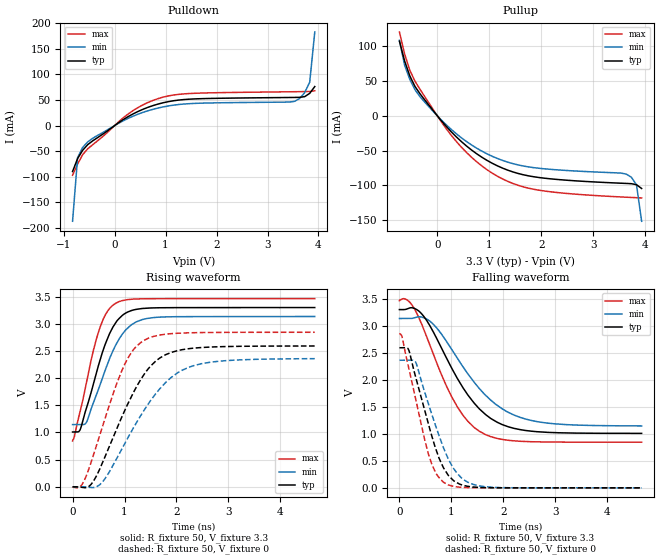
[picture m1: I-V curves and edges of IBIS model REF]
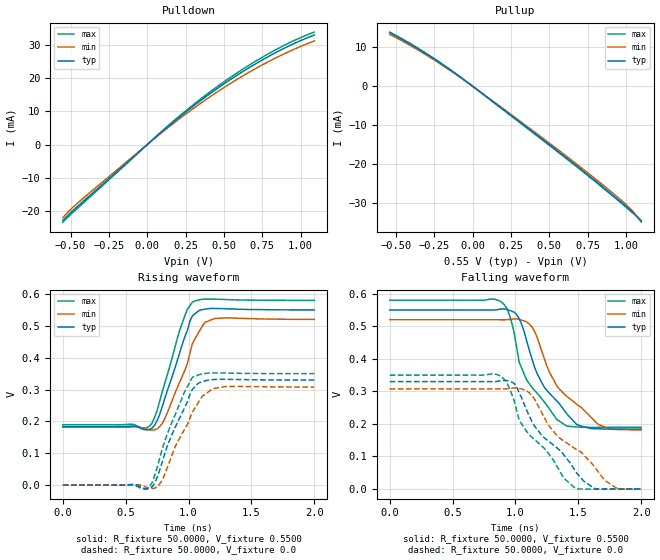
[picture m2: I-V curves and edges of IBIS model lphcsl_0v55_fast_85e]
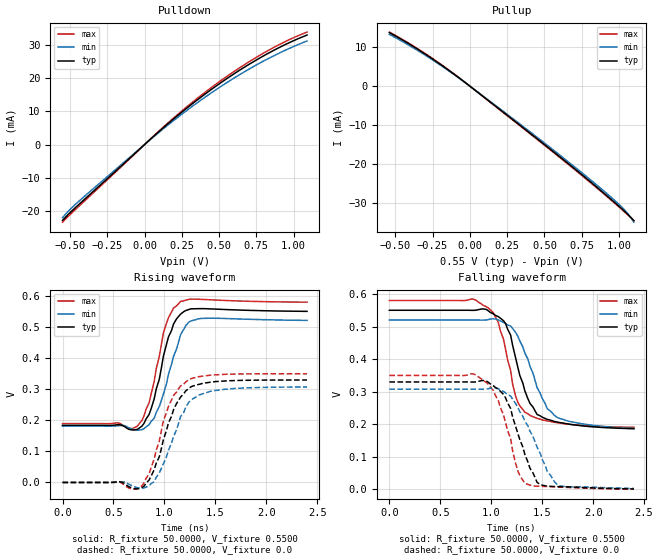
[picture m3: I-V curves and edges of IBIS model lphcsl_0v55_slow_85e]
| Integrated Devices Technolgy, Inc
[IBIS Ver]   4.1
[File name]   9fgl0651.ibs
[File Rev]   1.0
|Rev history   1.0   original ibis data
[Date]   30 March, 2016
[Disclaimer] Integrated Device Technology, Inc. ("IDT") hereby grants the
   user of this ibis model a non-exclusive, nontransferable
   license to use this ibis model under the following terms. the
   user is granted this license only to use the ibis model and is
   not granted rights to sell, copy (except as needed to run the
   ibis model), rent, lease or sub-license the ibis model in
   whole or in part, or in modified form to anyone. the user may
   modify the ibis model to suit its specific applications, but
   rights to derivative works and such modifications shall belong
   to idt. this ibis model is provided on an as is" basis and idt
   makes absolutely no warranty with respect to the information
   contained herein. idt disclaims and customer waives all
   warranties, express and implied, including warranties of
   merchantability and fitness for a particular purpose. the
   entire risk as to quality and performance is with the user
   accordingly, in no event shall idt be liable for any direct or
   indirect damages, whether in contract or tort, including any
   lost profits or other incidental, consequential, exemplary, or
   punitive damages arising out of the use or application of the
   ibis model. further, idt reserves the right to make changes
   without notice to any product herein to improve reliability,
   function, or design. idt does not convey any license under
   patent rights or any other intellectual property rights,
   including those of third parties. idt is not obligated to
   provide maintenance or support for the licensed ibis model.
[Copyright]   Copyright 2012, Integrated Devices Technolgy, Inc. all rights
   reserved
[Component]   9fgl0651
[Manufacturer] Integrated Device Technology, Inc.
[Package]
R_pkg   72.4655m   58.886m   86.045m
L_pkg   1.47175nH   1.11650nH   1.77850nH
C_pkg   0.07747pF   0.07444pF   0.08050pF
[Pin] signal_name  model_name
1   vSS_EN_tri   GND
2   X1_25   X1
3   X2   X2
4   VDDXTAL3.3   POWER
5   VDDREF3.3   POWER
6   vSADR/REF3.3   REF
7   NC   NC
8   GNDDIG   GND
9   SCLK_3.3   SCIN
10   SDATA_3.3   SCIN
11   VDDDIG3.3   POWER
12   VDDIO   POWER
13   vOE0#   IN
14   DIF0   LP_HCSL
15   DIF0#   LP_HCSL
16   VDD3.3   POWER
17   VDDIO   POWER
18   DIF1   LP_HCSL
19   DIF1#   LP_HCSL
20   NC   NC
21   vOE1#   IN
22   DIF2   LP_HCSL
23   DIF2#   LP_HCSL
24   vOE2#   IN
25   NC   NC
26   VDDA3.3   POWER
27   VDDIO   POWER
28   DIF3   LP_HCSL
29   DIF3#   LP_HCSL
30   vOE3#   IN
31   VDD3.3   POWER
32   VDDIO   POWER
33   DIF4   LP_HCSL
34   DIF4#   LP_HCSL
35   vOE4#   IN
36   DIF5   LP_HCSL
37   DIF5#   LP_HCSL
38   vOE5#   IN
39   VDDIO   POWER
40   ^CKPWRGD_PD#   PD
41   ePAD   GND
[Diff Pin]  inv_pin  vdiff tdelay_typ tdelay_min  tdelay_max
14   15   NA   0   0   0
18   19   NA   0   0   0
22   23   NA   0   0   0
28   29   NA   0   0   0
33   34   NA   0   0   0
36   37   NA   0   0   0
[Model Selector] LP_HCSL
lphcsl_0v55_fast_85e amplitude 0.55V, slew rate fast
lphcsl_0v55_slow_85e amplitude 0.55V, slew rate slow
lphcsl_0v65_fast_85e amplitude 0.65V, slew rate fast
lphcsl_0v65_slow_85e amplitude 0.65V, slew rate slow
lphcsl_0v70_fast_85e amplitude 0.70V, slew rate fast
lphcsl_0v70_slow_85e amplitude 0.70V, slew rate slow
lphcsl_0v80_fast_85e amplitude 0.80V, slew rate fast
lphcsl_0v80_slow_85e amplitude 0.80V, slew rate slow
| Models and submodels in the file (14): REF (Output), lphcsl_0v55_fast_85e (Output), lphcsl_0v55_slow_85e (Output), lphcsl_0v65_fast_85e (Output), lphcsl_0v65_slow_85e (Output), lphcsl_0v70_fast_85e (Output), lphcsl_0v70_slow_85e (Output), lphcsl_0v80_fast_85e (Output), lphcsl_0v80_slow_85e (Output), SCIN (Input), IN (Input), PD (Input), X1 (Input), X2 (Output)
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[Model]   REF
Model_type   Output
Polarity   Non-Inverting
|   typ   min   max
C_comp   2pF   1.5pF   2.5pF
Vmeas = 1.65V
Rref = 50
Cref = 0
Vref = 1.65V
|   typ   min   max
[Voltage range]   3.3V   3.135V   3.465V
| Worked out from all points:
|   slope of the pulldown table from 0 to 0.495 V, typ, clamps not added: 16.9 ohm
|   slope of the pullup table from 0 to 0.495 V, typ, clamps not added: 12.6 ohm
|   rising waveform, R_fixture 50, V_fixture 3.3: 20-80 % time 450ps typ, 507ps min, 388ps max; typ from 1.01 V to 3.3 V
|   falling waveform, R_fixture 50, V_fixture 3.3: 20-80 % time 857ps typ, 970ps min, 739ps max; typ from 3.3 V to 1.01 V
|   rising waveform, R_fixture 50, V_fixture 0: 20-80 % time 771ps typ, 936ps min, 618ps max; typ from 0 V to 2.59 V
|   falling waveform, R_fixture 50, V_fixture 0: 20-80 % time 472ps typ, 527ps min, 413ps max; typ from 2.59 V to 0 V
[Pulldown]
|Voltage   I (typ)   I (min)   I (max)
|Note, modeling breaks down at 250mA and above.  This is well beyond the functional   |
|operating range of the device.  Should this scenario occur, catastrophic failure and   |
|possible damage to the device and/or board is of higher concern than the I-V curve   |
|behavior.  The IBIS checker will flag currents in excess of 10A with warnings.  Lines   |
|with currents in excess of 0.35 A have been commented out.  The points still remain|
|available to the user if the user desires to use them.   |
|-3.30000e+00   -4.58626e+02   -3.98855e+02   -5.58913e+02
|-3.20100e+00   -4.38670e+02   -3.81813e+02   -5.34126e+02
|-3.10200e+00   -4.18718e+02   -3.64776e+02   -5.09343e+02
|-3.00300e+00   -3.98770e+02   -3.47745e+02   -4.84563e+02
|-2.90400e+00   -3.78827e+02   -3.30720e+02   -4.59787e+02
|-2.80500e+00   -3.58890e+02   -3.13701e+02   -4.35015e+02
|-2.70600e+00   -3.38959e+02   -2.96690e+02   -4.10248e+02
|-2.60700e+00   -3.19035e+02   -2.79688e+02   -3.85486e+02
|-2.50800e+00   -2.99119e+02   -2.62696e+02   -3.60731e+02
|-2.40900e+00   -2.79213e+02   -2.45715e+02   -3.35984e+02
|-2.31000e+00   -2.59319e+02   -2.28747e+02   -3.11245e+02
|-2.21100e+00   -2.39437e+02   -2.11796e+02   -2.86516e+02
|-2.11200e+00   -2.19572e+02   -1.94864e+02   -2.61800e+02
|-2.01300e+00   -1.99726e+02   -1.77955e+02   -2.37100e+02
|-1.91400e+00   -1.79905e+02   -1.61075e+02   -2.12419e+02
|-1.81500e+00   -1.60116e+02   -1.44233e+02   -1.87763e+02
|-1.71600e+00   -1.40369e+02   -1.27441e+02   -1.63140e+02
|-1.61700e+00   -1.20682e+02   -1.10717e+02   -1.38565e+02
|-1.51800e+00   -1.01080e+02   -9.40899e+01   -1.14061e+02
|-1.41900e+00   -8.16135e+01   -7.76121e+01   -8.96701e+01
|-1.32000e+00   -6.23864e+01   -6.13830e+01   -6.54941e+01
|-1.22100e+00   -4.36066e+01   -4.55730e+01   -4.17841e+01
|-1.12200e+00   -2.55446e+01   -3.03740e+01   -1.89497e+01
|-1.02300e+00   -8.13369e+00   -1.57511e+01   -1.01906e+00
|-9.24000e-01   -3.55892e-01   -2.38948e+00   -1.27879e-01
-825mV    -89.74mA   -186.9mA   -97.05mA
-726mV    -64.34mA   -62.46mA   -75.03mA
-627mV    -48.3mA    -42.65mA   -56.86mA
-528mV    -37.22mA   -31.89mA   -45.33mA
363mV     22.88mA    18.45mA    29.33mA
957mV     44.74mA    36.62mA    55.73mA
1.551V    52.05mA    43.3mA     63.04mA
3.531V    55.03mA    47.39mA    66.19mA
3.63V     55.21mA    52.95mA    66.32mA
3.729V    56.59mA    64.36mA    66.46mA
3.828V    63.02mA    84.81mA    66.64mA
3.927V    76.26mA    182.8mA    67.99mA
| 4.02600e+00   9.63336e-02   1.95544e+00   7.56685e-02
| 4.12500e+00   1.29319e-01   1.96109e+01   9.19025e-02
| 4.22400e+00   6.62462e-01   4.21550e+01   1.15435e-01
| 4.32300e+00   1.51637e+01   6.47670e+01   1.37492e-01
| 4.42200e+00   4.22442e+01   8.74545e+01   2.35006e-01
| 4.52100e+00   6.94172e+01   1.10195e+02   8.92943e+00
| 4.62000e+00   9.66780e+01   1.32968e+02   4.35589e+01
| 4.71900e+00   1.23991e+02   1.55761e+02   7.83218e+01
| 4.81800e+00   1.51333e+02   1.78569e+02   1.13180e+02
| 4.91700e+00   1.78693e+02   2.01386e+02   1.48085e+02
| 5.01600e+00   2.06065e+02   2.24210e+02   1.83014e+02
| 5.11500e+00   2.33446e+02   2.47041e+02   2.17958e+02
| 5.21400e+00   2.60834e+02   2.69877e+02   2.52912e+02
| 5.31300e+00   2.88228e+02   2.92717e+02   2.87874e+02
| 5.41200e+00   3.15625e+02   3.15560e+02   3.22841e+02
| 5.51100e+00   3.43027e+02   3.38407e+02   3.57813e+02
| 5.61000e+00   3.70432e+02   3.61256e+02   3.92789e+02
| 5.70900e+00   3.97841e+02   3.84108e+02   4.27769e+02
| 5.80800e+00   4.25252e+02   4.06963e+02   4.62752e+02
| 5.90700e+00   4.52666e+02   4.29821e+02   4.97738e+02
| 6.00600e+00   4.80082e+02   4.52680e+02   5.32727e+02
| 6.10500e+00   5.07501e+02   4.75543e+02   5.67718e+02
| 6.20400e+00   5.34922e+02   4.98407e+02   6.02711e+02
| 6.30300e+00   5.62345e+02   5.21273e+02   6.37705e+02
| 6.40200e+00   5.89770e+02   5.44142e+02   6.72701e+02
| 6.50100e+00   6.17197e+02   5.67013e+02   7.07699e+02
| 6.60000e+00   6.44626e+02   5.89886e+02   7.42698e+02
[Pullup]
|Voltage   I (typ)   I (min)   I (max)
|Note, modeling breaks down at 250mA and above.  This is well beyond the functional   |
|operating range of the device.  Should this scenario occur, catastrophic failure and   |
|possible damage to the device and/or board is of higher concern than the I-V curve   |
|behavior.  The IBIS checker will flag currents in excess of 10A with warnings.  Lines   |
|with currents in excess of 0.35 A have been commented out.  The points still remain|
|available to the user if the user desires to use them.   |
|-3.30000e+00   6.44680e+02   5.51825e+02   8.01095e+02
|-3.20100e+00   6.17254e+02   5.28958e+02   7.66095e+02
|-3.10200e+00   5.89830e+02   5.06093e+02   7.31096e+02
|-3.00300e+00   5.62407e+02   4.83230e+02   6.96098e+02
|-2.90400e+00   5.34987e+02   4.60368e+02   6.61102e+02
|-2.80500e+00   5.07568e+02   4.37509e+02   6.26108e+02
|-2.70600e+00   4.80150e+02   4.14651e+02   5.91115e+02
|-2.60700e+00   4.52735e+02   3.91796e+02   5.56124e+02
|-2.50800e+00   4.25322e+02   3.68942e+02   5.21136e+02
|-2.40900e+00   3.97911e+02   3.46091e+02   4.86149e+02
|-2.31000e+00   3.70503e+02   3.23243e+02   4.51165e+02
|-2.21100e+00   3.43097e+02   3.00397e+02   4.16183e+02
|-2.11200e+00   3.15694e+02   2.77554e+02   3.81204e+02
|-2.01300e+00   2.88295e+02   2.54715e+02   3.46229e+02
|-1.91400e+00   2.60900e+02   2.31881e+02   3.11257e+02
|-1.81500e+00   2.33510e+02   2.09052e+02   2.76290e+02
|-1.71600e+00   2.06127e+02   1.86229e+02   2.41329e+02
|-1.61700e+00   1.78751e+02   1.63415e+02   2.06375e+02
|-1.51800e+00   1.51388e+02   1.40613e+02   1.71432e+02
|-1.41900e+00   1.24042e+02   1.17829e+02   1.36506e+02
|-1.32000e+00   9.67252e+01   9.50724e+01   1.01609e+02
|-1.22100e+00   6.94599e+01   7.23604e+01   6.67700e+01
|-1.12200e+00   4.22820e+01   4.97173e+01   3.20469e+01
|-1.02300e+00   1.51962e+01   2.71494e+01   2.11287e+00
|-9.24000e-01   6.89030e-01   5.34223e+00   1.97623e-01
|-8.25000e-01   1.48916e-01   3.54714e-01   1.54087e-01
-726mV    106.9mA    108.2mA    120.1mA
-627mV    78.63mA    72.64mA    88.74mA
-528mV    57.36mA    52.3mA     65.5mA
-330mV    31.45mA    27.24mA    37.82mA
363mV     -30.02mA   -25.58mA   -36.52mA
957mV     -64.05mA   -54.65mA   -77.43mA
1.353V    -77.99mA   -66.51mA   -94.06mA
1.848V    -87.45mA   -74.38mA   -105.4mA
3.63V     -97.08mA   -83.63mA   -116.9mA
3.729V    -97.47mA   -88.18mA   -117.2mA
3.828V    -98.9mA    -99mA      -117.5mA
3.927V    -104.4mA   -151.4mA   -117.9mA
| 4.02600e+00   -1.15410e-01   -9.65481e-01   -1.19366e-01
| 4.12500e+00   -1.36603e-01   -1.09884e+01   -1.26324e-01
| 4.22400e+00   -3.99361e-01   -2.54841e+01   -1.40663e-01
| 4.32300e+00   -8.17474e+00   -4.04654e+01   -1.58277e-01
| 4.42200e+00   -2.55843e+01   -5.60873e+01   -2.17491e-01
| 4.52100e+00   -4.36450e+01   -7.21990e+01   -4.28595e+00
| 4.62000e+00   -6.24226e+01   -8.86071e+01   -2.64922e+01
| 4.71900e+00   -8.16508e+01   -1.05189e+02   -4.96573e+01
| 4.81800e+00   -1.01115e+02   -1.21884e+02   -7.35635e+01
| 4.91700e+00   -1.20715e+02   -1.38656e+02   -9.78285e+01
| 5.01600e+00   -1.40403e+02   -1.55482e+02   -1.22263e+02
| 5.11500e+00   -1.60149e+02   -1.72350e+02   -1.46794e+02
| 5.21400e+00   -1.79938e+02   -1.89250e+02   -1.71387e+02
| 5.31300e+00   -1.99760e+02   -2.06175e+02   -1.96022e+02
| 5.41200e+00   -2.19606e+02   -2.23121e+02   -2.20688e+02
| 5.51100e+00   -2.39472e+02   -2.40084e+02   -2.45378e+02
| 5.61000e+00   -2.59355e+02   -2.57061e+02   -2.70086e+02
| 5.70900e+00   -2.79251e+02   -2.74051e+02   -2.94808e+02
| 5.80800e+00   -2.99159e+02   -2.91052e+02   -3.19543e+02
| 5.90700e+00   -3.19077e+02   -3.08062e+02   -3.44288e+02
| 6.00600e+00   -3.39003e+02   -3.25080e+02   -3.69042e+02
| 6.10500e+00   -3.58937e+02   -3.42106e+02   -3.93803e+02
| 6.20400e+00   -3.78878e+02   -3.59138e+02   -4.18571e+02
| 6.30300e+00   -3.98826e+02   -3.76177e+02   -4.43346e+02
| 6.40200e+00   -4.18779e+02   -3.93221e+02   -4.68125e+02
| 6.50100e+00   -4.38737e+02   -4.10271e+02   -4.92910e+02
| 6.60000e+00   -4.58699e+02   -4.27325e+02   -5.17700e+02
[Ramp]
|   typ   min   max
dV/dt_r   1.566/0.774n   1.425/0.94n   1.718/0.621n
dV/dt_f   1.396/0.866n   1.212/0.979n   1.595/0.746n
R_load =   50
[Rising Waveform]
R_fixture = 50
V_fixture = 3.3   |Vcc_typ
V_fixture_min = 3.135 |Vcc_min
V_fixture_max = 3.465 |Vcc_max
C_fixture = 0.0p
| Time   typ   min   max
0s        1.008V     1.145V     844.6mV
34.71ps   1.008V     1.145V     923.1mV
154.3ps   1.071V     1.145V     1.413V
275.2ps   1.472V     1.202V     1.956V
479.5ps   2.168V     1.745V     2.789V
635.5ps   2.641V     2.166V     3.174V
823.7ps   3.01V      2.596V     3.375V
1.129ns   3.244V     2.981V     3.453V
1.433ns   3.289V     3.099V     3.463V
4.662ns   3.3V       3.135V     3.465V
[Falling Waveform]
R_fixture = 50
V_fixture = 3.3   |Vcc_typ
V_fixture_min = 3.135 |Vcc_min
V_fixture_max = 3.465 |Vcc_max
C_fixture = 0.0p
| Time   typ   min   max
0s        3.3V       3.135V     3.465V
120.3ps   3.304V     3.135V     3.493V
247.8ps   3.333V     3.138V     3.377V
425ps     3.225V     3.162V     3.038V
624.4ps   2.937V     3.054V     2.545V
1.111ns   2.034V     2.407V     1.506V
1.539ns   1.462V     1.838V     1.048V
1.979ns   1.171V     1.463V     896.3mV
2.515ns   1.052V     1.252V     854.4mV
4.666ns   1.008V     1.146V     844.6mV
[Rising Waveform]
R_fixture = 50
V_fixture = 0
C_fixture = 0.0p
| Time   typ   min   max
0s        23.89nV    60.43nV    30.4nV
191.1ps   -13.44mV   129.7uV    54.48mV
415.8ps   124mV      -13.01mV   625.4mV
623.1ps   548.9mV    147.1mV    1.254V
939.4ps   1.267V     680mV      2.117V
1.156ns   1.708V     1.059V     2.505V
1.348ns   2.027V     1.367V     2.681V
1.787ns   2.43V      1.916V     2.809V
2.339ns   2.554V     2.232V     2.838V
4.662ns   2.593V     2.359V     2.845V
[Falling Waveform]
R_fixture = 50
V_fixture = 0
C_fixture = 0.0p
| Time   typ   min   max
0s        2.593V     2.362V     2.845V
47.92ps   2.593V     2.362V     2.804V
169.8ps   2.571V     2.362V     2.258V
309ps     2.063V     2.332V     1.656V
482.9ps   1.445V     1.783V     905.2mV
624.2ps   958.6mV    1.36V      434.3mV
847.8ps   371.4mV    743.3mV    103.8mV
1.113ns   93.12mV    264.4mV    16.96mV
1.53ns    8.102mV    37.41mV    1.012mV
4.662ns   -1.039uV   -794nV     -867.7nV
[Model]   lphcsl_0v55_fast_85e
Model_type Output
Polarity   Inverting
Enable   Active-High
Vmeas =  0.4000V
Cref =   2.0000pF
Rref =   0.0
Vref =   0.4000V
C_comp   1.1000pF   1.0000pF   1.2000pF
[Temperature Range]   25.0000   85.0000   -40.0
[Voltage Range]   0.5500V   0.5200V   0.5800V
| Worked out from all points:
|   slope of the pulldown table from 0 to 0.083 V, typ, clamps not added: 24.5 ohm
|   slope of the pullup table from 0 to 0.083 V, typ, clamps not added: 33.4 ohm
|   rising waveform, R_fixture 50.0000, V_fixture 0.5500: 20-80 % time 183ps typ, 188ps min, 171ps max; typ from 0.184 V to 0.55 V
|   rising waveform, R_fixture 50.0000, V_fixture 0.0: 20-80 % time 207ps typ, 220ps min, 194ps max; typ from 0 V to 0.33 V
|   falling waveform, R_fixture 50.0000, V_fixture 0.5500: 20-80 % time 284ps typ, 342ps min, 253ps max; typ from 0.55 V to 0.184 V
|   falling waveform, R_fixture 50.0000, V_fixture 0.0: 20-80 % time 393ps typ, 449ps min, 348ps max; typ from 0.33 V to 0 V
[Pulldown]
|Voltage   I(typ)   I(min)   I(max)
-550mV    -22.86mA   -22.05mA   -23.4mA
-490mV    -20.12mA   -19.14mA   -20.7mA
-430mV    -17.63mA   -16.68mA   -18.17mA
50mV      2.058mA    1.922mA    2.135mA
230mV     9.045mA    8.465mA    9.373mA
410mV     15.37mA    14.42mA    15.91mA
590mV     21.04mA    19.77mA    21.74mA
770mV     26.03mA    24.5mA     26.86mA
930mV     29.87mA    28.16mA    30.76mA
1.09V     33.04mA    31.25mA    33.93mA
[Pullup]
|Voltage   I(typ)   I(min)   I(max)
-540mV    13.79mA    13.35mA    13.94mA
-360mV    9.757mA    9.424mA    9.891mA
-180mV    5.143mA    4.956mA    5.227mA
-20mV     596.4uA    573.5uA    607.4uA
340mV     -10.2mA    -9.898mA   -10.34mA
640mV     -19.35mA   -18.88mA   -19.54mA
920mV     -28.28mA   -27.72mA   -28.48mA
1.04V     -32.36mA   -32.02mA   -32.52mA
1.1V      -34.69mA   -35.06mA   -34.66mA
[Ramp]
| variable   typ   min   max
dV/dt_r  0.1979/0.2078n   0.1847/0.2401n   0.2100/0.1943n
dV/dt_f  0.2196/0.2840n   0.2029/0.3316n   0.2343/0.2729n
R_load = 50.0000
[Rising Waveform]
R_fixture= 50.0000
V_fixture= 0.5500
V_fixture_min= 0.5200
V_fixture_max= 0.5800
|time   V(typ)   V(min)   V(max)
0s        184mV      181.7mV    189.6mV
690ps     175.1mV    172.9mV    185.4mV
750ps     202.9mV    176.6mV    234.8mV
810ps     271.2mV    208.7mV    319.4mV
930ps     416.6mV    324.1mV    487.1mV
990ps     484.9mV    381.1mV    551.4mV
1.03ns    531.3mV    444mV      574.6mV
1.13ns    552.2mV    511mV      584.1mV
1.21ns    554.5mV    523.3mV    583.9mV
2ns       550mV      520.2mV    580mV
[Rising Waveform]
R_fixture= 50.0000
V_fixture= 0.0
V_fixture_min= 0.0
V_fixture_max= 0.0
|time   V(typ)   V(min)   V(max)
0s        0V         0V         0V
550ps     1.992mV    899.7uV    1.921mV
670ps     -12.01mV   -7.363mV   -11.15mV
730ps     6.349mV    -9.582mV   30.08mV
790ps     71.86mV    15.64mV    113.2mV
870ps     161.3mV    96.45mV    199.4mV
1.03ns    300.2mV    229mV      338.2mV
1.11ns    324.8mV    279.2mV    349.8mV
1.21ns    331.7mV    304.1mV    352.2mV
2ns       329.9mV    307.9mV    350mV
[Falling Waveform]
R_fixture= 50.0000
V_fixture= 0.5500
V_fixture_min= 0.5200
V_fixture_max= 0.5800
|time   V(typ)   V(min)   V(max)
0s        550mV      520mV      580mV
870ps     552mV      519.9mV    578.6mV
950ps     549mV      520.6mV    536.7mV
1.07ns    482.9mV    516.4mV    352.5mV
1.15ns    376.2mV    485.4mV    303.6mV
1.23ns    312.1mV    400.3mV    267mV
1.33ns    270.2mV    316.2mV    213.1mV
1.49ns    197.1mV    259.1mV    190.4mV
1.74ns    184.2mV    185.8mV    189.6mV
2ns       184mV      181.9mV    189.5mV
[Falling Waveform]
R_fixture= 50.0000
V_fixture= 0.0
V_fixture_min= 0.0
V_fixture_max= 0.0
|time   V(typ)   V(min)   V(max)
0s        329.9mV    307.7mV    349.9mV
870ps     331.7mV    307.6mV    349.1mV
990ps     324mV      310.6mV    270.6mV
1.07ns    260.1mV    304.5mV    187.9mV
1.15ns    194.6mV    276.9mV    152.6mV
1.33ns    126.2mV    164.2mV    69.85mV
1.47ns    59.22mV    125mV      4.447mV
1.54ns    25.17mV    106.1mV    -166.5uV
1.8ns     -314.8uV   3.333mV    -126.2uV
2ns       -24.85uV   -240.2uV   -19.95uV
[Model]   lphcsl_0v55_slow_85e
Model_type Output
Polarity   Inverting
Enable   Active-High
Vmeas =  0.4000V
Cref =   2.0000pF
Rref =   0.0
Vref =   0.4000V
C_comp   1.1000pF   1.0000pF   1.2000pF
[Temperature Range]   25.0000   85.0000   -40.0
[Voltage Range]   0.5500V   0.5200V   0.5800V
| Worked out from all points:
|   slope of the pulldown table from 0 to 0.083 V, typ, clamps not added: 24.5 ohm
|   slope of the pullup table from 0 to 0.083 V, typ, clamps not added: 33.4 ohm
|   rising waveform, R_fixture 50.0000, V_fixture 0.5500: 20-80 % time 164ps typ, 185ps min, 153ps max; typ from 0.184 V to 0.551 V
|   rising waveform, R_fixture 50.0000, V_fixture 0.0: 20-80 % time 212ps typ, 224ps min, 196ps max; typ from 0 V to 0.33 V
|   falling waveform, R_fixture 50.0000, V_fixture 0.5500: 20-80 % time 209ps typ, 258ps min, 182ps max; typ from 0.55 V to 0.186 V
|   falling waveform, R_fixture 50.0000, V_fixture 0.0: 20-80 % time 215ps typ, 272ps min, 192ps max; typ from 0.33 V to 0.002 V
[Pulldown]
|Voltage   I(typ)   I(min)   I(max)
-550mV    -22.86mA   -22.05mA   -23.4mA
-490mV    -20.12mA   -19.14mA   -20.7mA
-430mV    -17.63mA   -16.68mA   -18.17mA
50mV      2.058mA    1.922mA    2.135mA
230mV     9.045mA    8.465mA    9.373mA
410mV     15.37mA    14.42mA    15.91mA
590mV     21.04mA    19.77mA    21.74mA
770mV     26.03mA    24.5mA     26.86mA
930mV     29.87mA    28.16mA    30.76mA
1.09V     33.04mA    31.25mA    33.93mA
[Pullup]
|Voltage   I(typ)   I(min)   I(max)
-540mV    13.79mA    13.35mA    13.94mA
-360mV    9.757mA    9.424mA    9.891mA
-180mV    5.143mA    4.956mA    5.227mA
-20mV     596.4uA    573.5uA    607.4uA
340mV     -10.2mA    -9.898mA   -10.34mA
640mV     -19.35mA   -18.88mA   -19.54mA
920mV     -28.28mA   -27.72mA   -28.48mA
1.04V     -32.36mA   -32.02mA   -32.52mA
1.1V      -34.69mA   -35.06mA   -34.66mA
[Ramp]
| variable   typ   min   max
dV/dt_r  0.1981/0.2090n   0.1846/0.2327n   0.2101/0.1963n
dV/dt_f  0.2182/0.2310n   0.1998/0.2513n   0.2335/0.2061n
R_load = 50.0000
[Rising Waveform]
R_fixture= 50.0000
V_fixture= 0.5500
V_fixture_min= 0.5200
V_fixture_max= 0.5800
|time   V(typ)   V(min)   V(max)
0s        184mV      181.7mV    189.6mV
730ps     170.5mV    168.3mV    180.5mV
850ps     219.2mV    186.3mV    256.9mV
900ps     269.4mV    207.1mV    325.8mV
1.02ns    444.5mV    316.9mV    512.3mV
1.09ns    510.7mV    406.8mV    562.1mV
1.16ns    542.8mV    477.1mV    583.6mV
1.24ns    557.4mV    517mV      589.9mV
1.36ns    560.2mV    528.6mV    590.2mV
2.4ns     551.4mV    522.2mV    581mV
[Rising Waveform]
R_fixture= 50.0000
V_fixture= 0.0
V_fixture_min= 0.0
V_fixture_max= 0.0
|time   V(typ)   V(min)   V(max)
0s        0V         0V         0V
580ps     826.5uV    2.26mV     -2.284mV
700ps     -19.6mV    -13.42mV   -21.67mV
780ps     -16.64mV   -18.31mV   -10.91mV
900ps     41.24mV    2.869mV    75.98mV
1.04ns    192mV      104.4mV    244.9mV
1.12ns    254.6mV    169.8mV    291.5mV
1.24ns    302.9mV    258.8mV    331.7mV
1.55ns    326.1mV    298.5mV    347.8mV
2.4ns     330.1mV    307.6mV    350.1mV
[Falling Waveform]
R_fixture= 50.0000
V_fixture= 0.5500
V_fixture_min= 0.5200
V_fixture_max= 0.5800
|time   V(typ)   V(min)   V(max)
0s        550mV      520mV      580mV
820ps     549.7mV    520mV      584.4mV
1.07ns    530.3mV    520.6mV    512mV
1.19ns    473.7mV    501.6mV    365.3mV
1.24ns    402.5mV    481.5mV    285.3mV
1.33ns    302.2mV    418.6mV    237mV
1.45ns    230.1mV    312.6mV    218.2mV
1.55ns    215mV      247.5mV    210.2mV
1.65ns    206.8mV    220.7mV    204.8mV
2.4ns     186.4mV    187mV      190.8mV
[Falling Waveform]
R_fixture= 50.0000
V_fixture= 0.0
V_fixture_min= 0.0
V_fixture_max= 0.0
|time   V(typ)   V(min)   V(max)
0s        329.9mV    307.7mV    349.9mV
820ps     329.6mV    307.7mV    354.9mV
950ps     333.1mV    307.8mV    328.8mV
1.07ns    307.5mV    309.1mV    272mV
1.14ns    281.4mV    296.2mV    205.7mV
1.26ns    172.7mV    251.8mV    57.62mV
1.33ns    107.1mV    209.5mV    18.14mV
1.45ns    21.53mV    129.5mV    9.973mV
1.65ns    8.727mV    13.7mV     7.687mV
2.4ns     1.55mV     2.947mV    812.9uV
